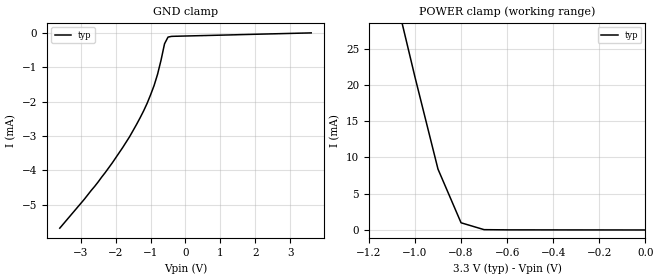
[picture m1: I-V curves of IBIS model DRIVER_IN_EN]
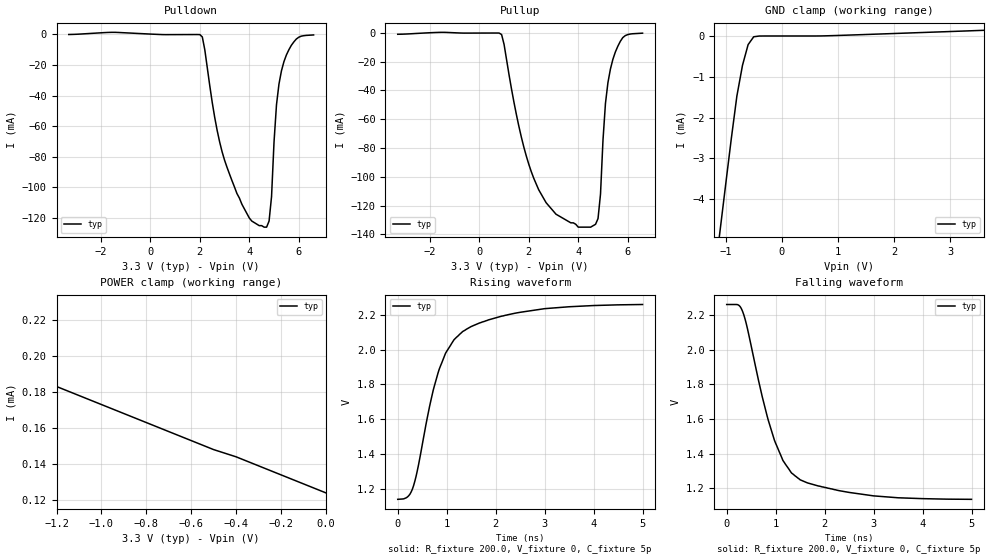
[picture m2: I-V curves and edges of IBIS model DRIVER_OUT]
|   Texas Instruments Incorporated
|   Data Transmissions Products
|   IBIS Model for TB5D2H
|   16DW SOIC Package
[IBIS Ver]   3.2
[Comment char]   |_char
[File name]   tb5d2h3v.ibs
[File Rev]   1.0
[Date]   14Apr03
[Source]   File originated at Texas Instruments Incorporated.
   Data Transmission Products Group. All data based on
   Simulation.
[Notes]  Model for 3V operation.
[Disclaimer]
(C) Copyright Texas Instruments Incorporated 2003
   All rights reserved
  Texas Instruments Incorporated hereby grants the user of this IBIS
model a non-exclusive, nontransferable license to use this IBIS model
under the following terms.  Before using this IBIS model, the user
should read this license.  If the user does not accept these terms,
the IBIS model should be returned to Texas Instruments within 30 days.
  The user is granted this license only to use the IBIS model and
is not granted rights to sell, load, rent, lease or license the IBIS
model in whole or in part, or in modified form to anyone other than
user.  User may modify the IBIS model to suit its specific applications
but rights to derivative works and such modifications shall belong to
Texas Instruments.
  This IBIS model is provided on an "AS IS" basis and Texas Instruments
makes absolutely no warranty with respect to the information contained
herein.  TEXAS INSTRUMENTS DISCLAIMS AND CUSTOMER WAIVES ALL WARRANTIES,
EXPRESS OR IMPLIED, INCLUDING WARRANTIES OF MERCHANTABILITY OR FITNESS
FOR A PARTICULAR PURPOSE. The entire risk as to quality and performance
is with the Customer. ACCORDINGLY, IN NO EVENT SHALL THE COMPANY BE LIABLE
FOR ANY DAMAGES, WHETHER IN CONTRACT OR TORT,INCLUDING ANY LOST PROFITS
OR OTHER INCIDENTAL, CONSEQUENTIAL, EXEMPLARY, OR PUNITIVE DAMAGES ARISING
OUT OF THE USE OR APPLICATION OF THE IBIS model provided in this package.
Further, Texas Instruments reserves the right to discontinue or make changes
without notice to any product herein to improve reliability, function, or
design. Texas Instruments does not convey any license under patent rights
or any other intellectual property rights, including those of third parties.
Contact Texas Instruments at ATTN:DATA TRANSMISSIONS
[Copyright]   Copyright 2003, Texas Instruments, All Rights Reserved
[Component]   TB5D2H
[Manufacturer]  Texas Instruments
[Package]
|   typ   min   max
R_pkg   0.046   0.034   0.057
L_pkg   4.858nH   3.987nH   6.214nH
C_pkg   0.715pF   0.502pF   1.046pF
[Pin]   signal_name   model_name   R_pin   L_pin   C_pin
1   AI   DRIVER_IN_EN   0.057   6.214nH   1.026pF
2   AO   DRIVER_OUT   0.055   5.236nH   0.818pF
3   AO(-)   DRIVER_OUT   0.034   3.987nH   0.723pF
4   E1   DRIVER_IN_EN   0.036   3.996nH   0.726pF
5   BO(-)   DRIVER_OUT   0.036   3.996nH   0.726pF
6   BO   DRIVER_OUT   0.034   3.987nH   0.704pF
7   BI   DRIVER_IN_EN   0.055   5.236nH   0.818pF
8   GND   GND   0.057   6.214nH   1.046pF
9   CI   DRIVER_IN_EN   0.057   6.214nH   0.827pF
10   CO   DRIVER_OUT   0.055   5.236nH   0.597pF
11   CO(-)   DRIVER_OUT   0.034   3.987nH   0.502pF
12   E2   DRIVER_IN_EN   0.036   3.996nH   0.505pF
13   DO(-)   DRIVER_OUT   0.036   3.996nH   0.505pF
14   DO   DRIVER_OUT   0.034   3.987nH   0.502pF
15   DI   DRIVER_IN_EN   0.055   5.236nH   0.597pF
16   VCC   POWER   0.057   6.214nH   0.827pF
[Diff_pin]   inv_pin   vdiff   tdelay_typ   tdelay_min   tdelay_max
| The 'AO(+) (or 'xO(+)')' and inv_pins, 'AO(-) (or 'xO(-)')', pins
| are Diff_pins
   2   3   0   0   0   0
   6   5   0   0   0   0
   10   11   0   0   0   0
   14   13   0   0   0   0
| Models and submodels in the file (2): DRIVER_IN_EN (Input), DRIVER_OUT (Output_ECL)
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|   Driver Input Model
[Model]   DRIVER_IN_EN
Model_type   Input
|Signals   AI,BI,CI,DI,E1,E2
Vinh = 2.4
Vinl = 0.4
|   typ   min   max
C_comp   1.03pF   NA   NA
|   typ   min   max
[Temperature Range]   25.0   NA   NA
[Voltage range]   3.3V   NA   NA
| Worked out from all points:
|   GND clamp passes 1 mA (typ) near -0.75 V on its own axis
|   POWER clamp passes 1 mA (typ) near -0.80 V on its own axis
[GND_clamp]
| Voltage   I(typ)   I(min)   I(max)
-3.6V     -5.69mA    NA         NA
-2.5V     -4.34mA    NA         NA
-2.1V     -3.79mA    NA         NA
-1.6V     -3.02mA    NA         NA
-1.2V     -2.27mA    NA         NA
-1V       -1.8mA     NA         NA
-900mV    -1.53mA    NA         NA
-800mV    -1.2mA     NA         NA
-700mV    -787uA     NA         NA
-600mV    -309uA     NA         NA
-500mV    -114uA     NA         NA
3.6V      8.57uA     NA         NA
[Power_clamp]
| Note that the[POWER_clamp]voltage table is referenced to Vcc
| and is calculated using Vtable=Vcc - Vmeasured.
|   Voltage   I(typ)   I(min)   I(max)
-3.3V     147mA      NA         NA
-1.1V     34.4mA     NA         NA
-1V       21.1mA     NA         NA
-900mV    8.39mA     NA         NA
-800mV    993uA      NA         NA
-700mV    43.8uA     NA         NA
0V        1.05uA     NA         NA
|   Driver Output Model
[Model]   DRIVER_OUT
|Model_type   3-state_ECL
Model_type   Output_ECL
| Signals   O(+),O(-)
Vmeas = 1.8V   |Reference voltage for timing measurements
Cref = 5pF   |Timing specification test load capacitance value
Rref = 200   |Note: 200 Ohm load; single ended configuration
| variable   typ   min   max
C_comp   920fF   NA   NA
|   typ   min   max
[Temperature Range]   25.0   NA   NA
[Voltage range]   3.3V   NA   NA
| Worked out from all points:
|   GND clamp passes 1 mA (typ) near -0.74 V on its own axis
|   POWER clamp passes 1 mA (typ) near -1.97 V on its own axis
|   rising waveform, R_fixture 200.0, V_fixture 0, C_fixture 5p: 20-80 % time 659ps typ, NA min, NA max; typ from 1.14 V to 2.26 V
|   falling waveform, R_fixture 200.0, V_fixture 0, C_fixture 5p: 20-80 % time 658ps typ, NA min, NA max; typ from 2.26 V to 1.14 V
[Pulldown]
|   Voltage   I(typ)   I(min)   I(max)
-3.3V     -6uA       NA         NA
2.1V      -1.6mA     NA         NA
2.6V      -54.1mA    NA         NA
3V        -82.2mA    NA         NA
4V        -120mA     NA         NA
4.6V      -126mA     NA         NA
4.8V      -122mA     NA         NA
4.9V      -106mA     NA         NA
5.1V      -45.9mA    NA         NA
5.3V      -23.8mA    NA         NA
5.9V      -3mA       NA         NA
6.6V      -300uA     NA         NA
[Pullup]
|   Voltage   I(typ)   I(min)   I(max)
| Note that the[Pullup]voltage table is referenced to Vcc
| and is calculated using Vtable=Vcc - Vmeasured.
-3.3V     -965uA     NA         NA
900mV     -1.15mA    NA         NA
1.7V      -72.5mA    NA         NA
2.4V      -109mA     NA         NA
3.1V      -126mA     NA         NA
4.5V      -135mA     NA         NA
4.8V      -129mA     NA         NA
4.9V      -112mA     NA         NA
5.1V      -49mA      NA         NA
5.4V      -18.4mA    NA         NA
5.8V      -3.3mA     NA         NA
6.6V      -200uA     NA         NA
[GND_clamp]
|   Voltage   I(typ)   I(min)   I(max)
| Outputs in High Impedance (off)
-3.6V     -165mA     NA         NA
-1.1V     -4.77mA    NA         NA
-900mV    -2.52mA    NA         NA
-800mV    -1.47mA    NA         NA
-700mV    -718uA     NA         NA
-600mV    -212uA     NA         NA
-500mV    -19.1uA    NA         NA
-400mV    -976nA     NA         NA
800mV     4.54uA     NA         NA
3.6V      139uA      NA         NA
[Power_clamp]
| Note that the[POWER_clamp]voltage table is referenced to Vcc
| and is calculated using Vtable=Vcc - Vmeasured.
|   Voltage   I(typ)   I(min)   I(max)
-3.3V     3.59mA     NA         NA
-1.5V     281uA      NA         NA
-1.4V     214uA      NA         NA
-1.3V     190uA      NA         NA
-1.2V     183uA      NA         NA
-500mV    148uA      NA         NA
-400mV    144uA      NA         NA
0V        124uA      NA         NA
[Ramp]
|   typ   min   max
dV/dt_r   0.676/663ps   NA   NA
dV/dt_f   0.676/658ps   NA   NA
R_load = 200ohm
[Rising Waveform]
R_fixture = 200.0
V_fixture = 0
C_fixture = 5p
|   V(typ)   V(min)   V(max)
0s        1.138V     NA         NA
175ps     1.147V     NA         NA
300ps     1.197V     NA         NA
400ps     1.303V     NA         NA
675ps     1.705V     NA         NA
825ps     1.868V     NA         NA
1ns       1.991V     NA         NA
1.325ns   2.105V     NA         NA
2.5ns     2.216V     NA         NA
5ns       2.261V     NA         NA
[Falling Waveform]
R_fixture = 200.0
V_fixture = 0
C_fixture = 5p
|   V(typ)   V(min)   V(max)
0s        2.262V     NA         NA
225ps     2.261V     NA         NA
325ps     2.222V     NA         NA
725ps     1.73V      NA         NA
975ps     1.477V     NA         NA
1.15ns    1.359V     NA         NA
1.4ns     1.27V      NA         NA
1.875ns   1.212V     NA         NA
3ns       1.155V     NA         NA
5ns       1.135V     NA         NA
